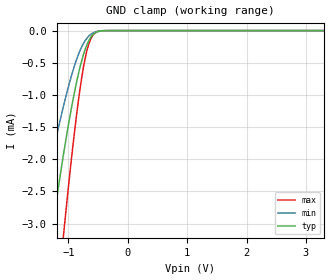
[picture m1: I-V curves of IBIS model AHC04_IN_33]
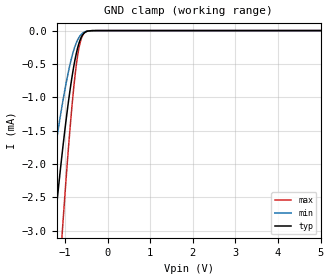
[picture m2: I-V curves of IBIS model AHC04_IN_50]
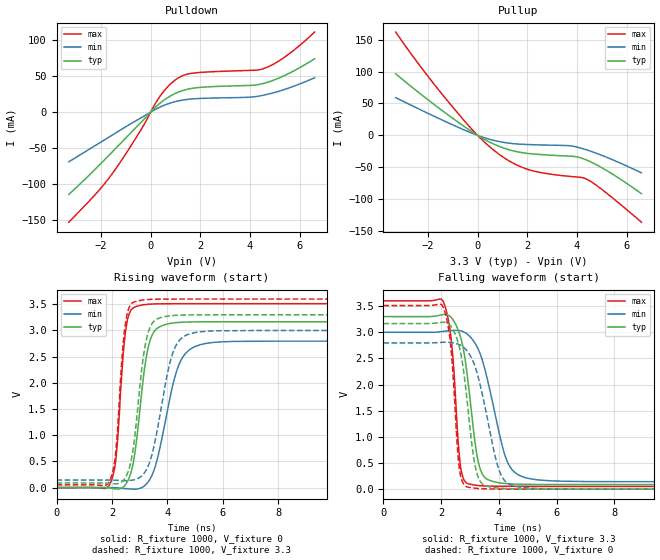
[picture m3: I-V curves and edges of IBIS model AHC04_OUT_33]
| TEXAS INSTRUMENTS INCORPORATED
| Standard Linear and Logic Group
| IBIS Model of SN54AHC04
| HEX INVERTERS
| This file contains package information for the following:
| This device can be powered at the following Vccs:
|  3.3 volt Vcc
|  5 volt Vcc
| This file provides unique models under the [Model Selector] for each Vcc.
| For operation at a specific Vcc, select the appropriate model after each
| [Model Selector] keyword.
[IBIS Ver]   3.2
[Comment char]  |_char
[File Name]   sn54ahcu04.ibs
[File Rev]   1.1 | b_die
[Date]   May 16, 2003
[Source]   Data created from TI-SPICE simulations at TI-SLL.
[Notes]   The following is an IBIS list for the AHC04.
   Please contact sllibis@ti.com with questions and
   comments concerning SLL IBIS models.
   This IBIS model is created from a BA (back annotated
   netlist).
   - Power-clamp data has been deleted from the input model
   Dec 13, 2009
   Modified SN74 model to create ceramic SN54 model
[Disclaimer] Property of Texas Instruments Incorporated.  Unauthorized
   reproduction and/or distribution is strictly prohibited.
   This product is protected under copyright law.
   Created  2003, (C) Copyright  2003, Texas Instruments
   Incorporated, All Rights Reserved
   UNLESS THERE IS A SIGNED, WRITTEN AGREEMENT TO THE
   CONTRARY, TEXAS INSTRUMENTS (TI) IS PROVIDING THE IBIS
   MODELS  AND WITHOUT ANY WARRANTY, EXPRESSED OR
   IMPLIED.  TI assumes no liability for:
   1) the accuracy of the IBIS models provided to your
   company;
   2) the proper functioning of these IBIS Models in your
   design or for any resulting applications; or
   3) infringement of patents, copyrights or intellectual
   property rights resulting from your use of these IBIS
   models.
   TI provides IBIS Models as a service to our customers.
   You and your company shall not distribute, sell or give
   these models to anyone else without prior written
   permission from TI.
   TI reserves the right to make changes to our products or
   to discontinue any semiconductor product or service
   without notice, and advises our customers to obtain the
   latest version of relevant information to verify, before
   placing orders, that the information being relied on is
   current.
   Please be aware that your receipt and use of the IBIS
   information provided shall serve as acceptance of these
   terms and conditions.  If you do not accept these terms,
   you should return or destroy the IBIS models and any
   other accompanying information immediately.
| Component AHC04_W 14-pin
[Component]   AHC04_W
[Manufacturer]   Texas Instruments, Inc.
[Package]
|   typ   min   max
R_pkg   0.091   0.077   0.111
L_pkg   5.063e-9   4.367e-9   6.264e-9
C_pkg   1.809e-12  1.649e-12   2.160e-12
[Pin]   signal_name   model_name   R_pin   L_pin   C_pin
1   1A   AHC04_IN   0.106   6.098e-9 2.108e-12
2   1Y   AHC04_OUT   0.087   4.760e-9 1.771e-12
3   2A   AHC04_IN   0.078   4.393e-9 1.649e-12
4   2Y   AHC04_OUT   0.077   4.367e-9 1.650e-12
5   3A   AHC04_IN   0.085   4.675e-9 1.709e-12
6   3Y   AHC04_OUT   0.090   4.850e-9 1.678e-12
7   GND   GND   0.111   6.264e-9 2.160e-12
8   4Y   AHC04_OUT   0.110   6.228e-9 2.146e-12
9   4A   AHC04_IN   0.093   4.955e-9 1.700e-12
10   5Y   AHC04_OUT   0.080   4.501e-9 1.687e-12
11   5A   AHC04_IN   0.077   4.371e-9 1.655e-12
12   6Y   AHC04_OUT   0.083   4.610e-9 1.705e-12
13   6A   AHC04_IN   0.086   4.701e-9 1.657e-12
14   VCC   POWER   0.107   6.111e-9 2.055e-12
| Model AHC04_IN
[Model Selector]   AHC04_IN
AHC04_IN_33   3.3 volt Vcc
AHC04_IN_50   5 volt Vcc
| Model AHC04_OUT
[Model Selector]   AHC04_OUT
AHC04_OUT_33   3.3 volt Vcc
AHC04_OUT_50   5 volt Vcc
| Models and submodels in the file (4): AHC04_IN_33 (Input), AHC04_IN_50 (Input), AHC04_OUT_33 (Output), AHC04_OUT_50 (Output)
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[Model]   AHC04_IN_33
Model_type  Input
Vinl = 0.9
Vinh = 2.1
| variable   typ   min   max
C_comp   0.64pF   0.52pF   0.73pF
[Temperature Range]   40   100   -40
| Ambient temperature   25   85   -40
[Voltage range]   3.3   3   3.6
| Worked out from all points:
|   GND clamp passes 1 mA (typ) near -0.91 V on its own axis
[GND Clamp]
| AHC04_IN_33
|   Voltage   I(typ)   I(min)   I(max)
-3.3V     -21.05mA   -13.78mA   -28.64mA
-1.52V    -4.845mA   -3.097mA   -7.647mA
-1.28V    -3.152mA   -1.983mA   -5.117mA
-1.1V     -2.026mA   -1.24mA    -3.347mA
-1.07V    -1.853mA   -1.126mA   -3.066mA
-905mV    -992.8uA   -568.6uA   -1.638mA
-835mV    -688.4uA   -381uA     -1.115mA
-770mV    -449.4uA   -241.7uA   -699.2uA
-675mV    -193uA     -104uA     -265.9uA
-575mV    -52.68uA   -32.06uA   -58.42uA
-375mV    -1.402uA   -1.027uA   -717.1nA
3.3V      3.885nA    645.3pA    18.64nA
[Model]   AHC04_IN_50
Model_type  Input
Vinl = 1.65
Vinh = 3.85
| variable   typ   min   max
C_comp   0.63pF   0.51pF   0.74pF
[Temperature Range]   40   100   -40
| Ambient temperature   25   85   -40
[Voltage range]   5   4.5   5.5
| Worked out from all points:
|   GND clamp passes 1 mA (typ) near -0.91 V on its own axis
[GND Clamp]
| AHC04_IN_50
|   Voltage   I(typ)   I(min)   I(max)
-5V       -39.11mA   -25.77mA   -50.08mA
-1.5V     -4.697mA   -2.999mA   -7.43mA
-1.27V    -3.086mA   -1.94mA    -5.015mA
-1.245V   -2.922mA   -1.832mA   -4.762mA
-1.07V    -1.853mA   -1.126mA   -3.066mA
-1.05V    -1.74mA    -1.052mA   -2.883mA
-875mV    -857.1uA   -483.9uA   -1.406mA
-765mV    -433uA     -232.5uA   -670.7uA
-665mV    -173.1uA   -93.8uA    -234.3uA
-615mV    -93.6uA    -53.56uA   -114.5uA
-545mV    -32.78uA   -20.83uA   -33.46uA
5V        15.07nA    1.006nA    138.2nA
[Model]   AHC04_OUT_33
Model_type  Output
Vref =   0
Rref =   1000
Cref =   50p
Vmeas =   1.65
| variable   typ   min   max
C_comp   2.86pF   1.54pF   4.00pF
| C_pullup   2.82pF   1.54pF   3.49pF
| C_pulldown   2.90pF   1.77pF   4.00pF
[Temperature Range]   40   100   -40
| Ambient temperature   25   85   -40
[Voltage range]   3.3   3   3.6
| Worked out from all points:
|   slope of the pulldown table from 0 to 0.495 V, typ, clamps not added: 31.8 ohm
|   slope of the pullup table from 0 to 0.495 V, typ, clamps not added: 45.8 ohm
|   rising waveform, R_fixture 1000, V_fixture 0: 20-80 % time 434ps typ, 700ps min, 283ps max; typ from 0 V to 3.17 V
|   falling waveform, R_fixture 1000, V_fixture 3.3: 20-80 % time 439ps typ, 727ps min, 267ps max; typ from 3.3 V to 0.088 V
|   rising waveform, R_fixture 1000, V_fixture 3.3: 20-80 % time 418ps typ, 632ps min, 279ps max; typ from 0.088 V to 3.3 V
|   falling waveform, R_fixture 1000, V_fixture 0: 20-80 % time 419ps typ, 665ps min, 255ps max; typ from 3.17 V to 0 V
[Pulldown]
| AHC04_OUT_33
|   Voltage   I(typ)   I(min)   I(max)
-3.3V     -114.4mA   -69.04mA   -152.9mA
-2.22V    -78.8mA    -46.22mA   -113.9mA
-1.635V   -58.39mA   -33.79mA   -89.51mA
-480mV    -17.44mA   -9.793mA   -29.54mA
330mV     11.04mA    6.164mA    19.74mA
635mV     18.98mA    10.63mA    33.32mA
955mV     25.27mA    14.14mA    43.64mA
1.295V    29.94mA    16.67mA    50.63mA
1.685V    33.04mA    18.27mA    53.93mA
4.555V    39.87mA    23.49mA    60.41mA
5.45V     51.66mA    32.05mA    77.66mA
6.6V      73.99mA    47.56mA    111mA
[Pullup]
| AHC04_OUT_33
|   Voltage   I(typ)   I(min)   I(max)
-3.3V     96.43mA    59.11mA    161.8mA
-2.19V    61.53mA    38.04mA    102.2mA
-995mV    26.52mA    16.31mA    43.97mA
-15mV     367.5uA    219.4uA    603.7uA
745mV     -15.3mA    -8.685mA   -26.19mA
1.415V    -24.13mA   -12.91mA   -43.25mA
2.085V    -28.58mA   -14.44mA   -54.08mA
3.69V     -32.57mA   -16.26mA   -64.18mA
4.03V     -33.95mA   -18.66mA   -65.36mA
4.39V     -38.7mA    -22.73mA   -68.57mA
5.315V    -57.85mA   -36.24mA   -94.18mA
6.6V      -91.36mA   -58.68mA   -136.1mA
[Ramp]
| AHC04_OUT_33
| variable   typ   min   max
dV/dt_r   1.92/4.43E-10   1.70/7.09E-10   2.12/2.98E-10
dV/dt_f   1.95/4.54E-10   1.74/7.41E-10   2.15/2.80E-10
R_load = 1000
[Rising Waveform]
| AHC04_OUT_33
R_fixture =   1000
C_fixture =   0
L_fixture =   0
V_fixture =   0
V_fixture_min = 0
V_fixture_max = 0
|   Time   V(typ)   V(min)   V(max)
0s        923.7pV    1.562nV    526.1pV
1.94ns    -10.94mV   922.7uV    79.68mV
2.15ns    -26.28mV   -3.1mV     589.2mV
2.545ns   101.3mV    -22.73mV   3.159V
2.815ns   610.7mV    -30.5mV    3.445V
3.155ns   2.186V     25.06mV    3.492V
3.53ns    2.984V     346.5mV    3.507V
4.465ns   3.155V     2.401V     3.511V
5.6ns     3.166V     2.769V     3.511V
50ns      3.167V     2.797V     3.511V
[Falling Waveform]
| AHC04_OUT_33
R_fixture =   1000
C_fixture =   0
L_fixture =   0
V_fixture =   3.3
V_fixture_min = 3
V_fixture_max = 3.6
|   Time   V(typ)   V(min)   V(max)
0s        3.3V       3V         3.6V
2.07ns    3.338V     3.017V     3.585V
2.355ns   3.28V      3.033V     2.824V
2.595ns   3.032V     3.034V     858.1mV
2.69ns    2.869V     3.026V     367.8mV
3.225ns   698.1mV    2.74V      73.16mV
3.51ns    222.2mV    2.3V       61.01mV
4.31ns    104.6mV    504mV      53.79mV
5.385ns   89.79mV    175.3mV    52.7mV
50ns      87.98mV    143.4mV    52.56mV
[Rising Waveform]
| AHC04_OUT_33
R_fixture =   1000
C_fixture =   0
L_fixture =   0
V_fixture =   3.3
V_fixture_min = 3
V_fixture_max = 3.6
|   Time   V(typ)   V(min)   V(max)
0s        87.98mV    143.4mV    52.56mV
1.925ns   79.6mV     143.7mV    133.8mV
2.13ns    72.37mV    140.4mV    638.1mV
2.52ns    223.7mV    131.9mV    3.237V
2.765ns   732.8mV    144.8mV    3.534V
3.115ns   2.421V     243.6mV    3.582V
3.465ns   3.144V     673.1mV    3.595V
4.235ns   3.287V     2.622V     3.6V
5.2ns     3.299V     2.976V     3.6V
50ns      3.3V       3V         3.6V
[Falling Waveform]
| AHC04_OUT_33
R_fixture =   1000
C_fixture =   0
L_fixture =   0
V_fixture =   0
V_fixture_min = 0
V_fixture_max = 0
|   Time   V(typ)   V(min)   V(max)
0s        3.167V     2.797V     3.511V
2.065ns   3.192V     2.809V     3.483V
2.325ns   3.123V     2.805V     2.775V
2.63ns    2.718V     2.763V     398.7mV
3ns       1.167V     2.561V     30.42mV
3.15ns    523.1mV    2.382V     20.62mV
3.315ns   186.7mV    2.071V     12.06mV
4.04ns    17.32mV    313.1mV    1.945mV
4.905ns   2.668mV    27.01mV    339uV
50ns      -13.44nV   -7.509nV   -6.235nV
